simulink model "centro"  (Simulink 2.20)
settings: Solver=VariableStepDiscrete  StartTime=0.0  StopTime=40.0  RelTol=1e-3  AbsTol=1e-6
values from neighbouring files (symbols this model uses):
  a = input('Inserisci il dato da graficare [1=PIDNL 2=PD 3=PID]: ')    [grp.m]    (also in grp1.m = input('Inserisci il dato da graficare [1..3]'))
undefined symbols (not defined in the file or in its folder): b
libraries: Puma x3, simulink x3

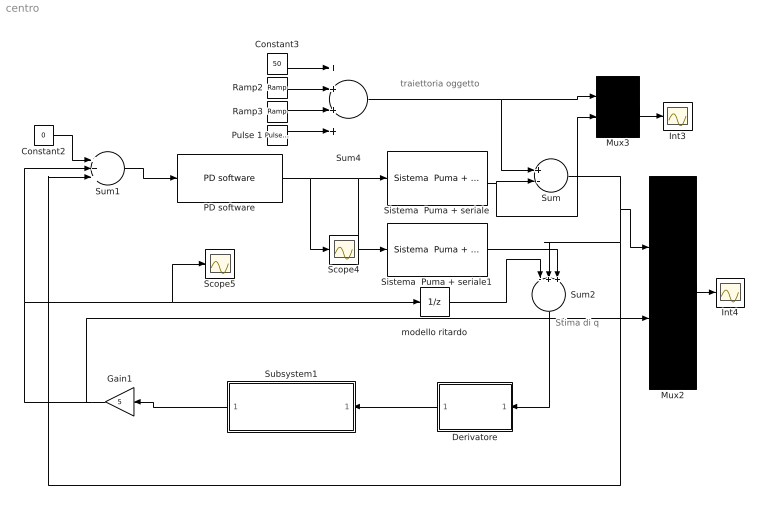
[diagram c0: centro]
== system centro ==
  note: Stima di q
  note: traiettoria oggetto
  Constant2 : Constant  Value=0
  Constant3 : Constant  Value=50
  Derivatore : Subsystem  Orientation=left  mask(Simulazione Derivatore implementato in maniera software){Td=0.13, T=0.40, N=5}
      mask prompts: Td "Costante di derivazione Td"; T "Sample Time T del PD"; N "Indice polo del derivatore [5..10]"
      mask init:
      | Kbeta=Td/(N*T+Td);
      | Kalfa=N*Kbeta;
  Gain1 : Gain  Orientation=left  Gain=5
  Int3 : Scope
  Int4 : Scope
  Mux2 : Mux  Inputs=2
  Mux3 : Mux  Inputs=2
  PD software : Puma/PD software  Kp=0.5  Td=0.1  T=0.130  N=10
  Pulse 1 : simulink/Sources/Pulse Generator  period=30  duty=10  amplitude=-50  start=30
  Ramp2 : simulink/Sources/Ramp  slope=-50  start=10  X0=0
  Ramp3 : simulink/Sources/Ramp  slope=+50  start=25  X0=0
  Scope4 : Scope
  Scope5 : Scope
  Sistema  Puma + seriale : Puma/Sistema  Puma + seriale  Ts=.260
  Sistema  Puma + seriale1 : Puma/Sistema  Puma + seriale  Ts=.260
  Subsystem1 : Subsystem  Orientation=left  mask(Filtro di Butterworth){ordine=1, freq=0.1/16}
      mask prompts: ordine "Ordine del filtro"; freq "Parametro K per ricavare la Freq. di taglio Ft"
      mask help: Attenzione! Considerare il parametro Fc come la frequanza di campionamento del segnale di ingresso, per cui la frequanza di taglio diviene Ft=K*Fc;
      mask init:
      | [b,a]=butter(ordine,freq);
  Sum : Sum  Inputs=+-
  Sum1 : Sum  Inputs=+++
  Sum2 : Sum  Orientation=down  Inputs=-++
  Sum4 : Sum  Inputs=++++
  modello ritardo : UnitDelay  X0=0  SampleTime=.320
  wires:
  Mux2/1 -> Int4/1
  Sistema  Puma + seriale/1 -> Sum/2, Mux3/2
  Sum2/1 -> Derivatore/1(In1)
  Sum/1 -> Mux2/1, Sum2/2, Sum1/3
  Mux3/1 -> Int3/1
  Gain1/1 -> Mux2/2, modello ritardo/1, Scope5/1, Sum1/2
  Sum1/1 -> PD software/1
  PD software/1 -> Sistema  Puma + seriale/1, Sistema  Puma + seriale1/1, Scope4/1
  modello ritardo/1 -> Sum2/1
  Sistema  Puma + seriale1/1 -> Sum2/3
  Constant2/1 -> Sum1/1
  Derivatore/1(Out1) -> Subsystem1/1(In1)
  Subsystem1/1(Out1) -> Gain1/1
  Pulse 1/1 -> Sum4/4
  Constant3/1 -> Sum4/1
  Ramp2/1 -> Sum4/2
  Ramp3/1 -> Sum4/3
  Sum4/1 -> Mux3/1, Sum/1

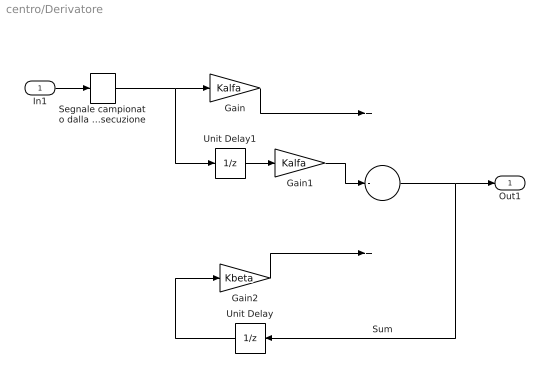
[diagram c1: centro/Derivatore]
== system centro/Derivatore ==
  In1 : Inport  Port=1  PortWidth=-1  SampleTime=-1
  Gain : Gain  Gain=Kalfa
  Gain1 : Gain  Gain=Kalfa
  Gain2 : Gain  Gain=Kbeta
  Segnale campionato dalla procedura software al momento del ciclo  d 'esecuzione : ZeroOrderHold  SampleTime=T
  Sum : Sum  Inputs=+-+
  Unit Delay : UnitDelay  Orientation=left  X0=0  SampleTime=T
  Unit Delay1 : UnitDelay  X0=0  SampleTime=T
  Out1 : Outport  Port=1
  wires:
  Gain1/1 -> Sum/2
  Unit Delay/1 -> Gain2/1
  Gain2/1 -> Sum/3
  Gain/1 -> Sum/1
  Unit Delay1/1 -> Gain1/1
  Sum/1 -> Out1/1, Unit Delay/1
  In1/1 -> Segnale campionato dalla procedura software al momento del ciclo  d 'esecuzione/1
  Segnale campionato dalla procedura software al momento del ciclo  d 'esecuzione/1 -> Gain/1, Unit Delay1/1

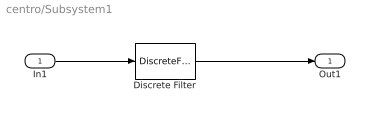
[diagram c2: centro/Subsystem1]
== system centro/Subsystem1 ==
  In1 : Inport  Port=1  PortWidth=-1  SampleTime=-1
  Discrete Filter : DiscreteFilter  Numerator=b  Denominator=a  SampleTime=.032
  Out1 : Outport  Port=1
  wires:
  In1/1 -> Discrete Filter/1
  Discrete Filter/1 -> Out1/1
